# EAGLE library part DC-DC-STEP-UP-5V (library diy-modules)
DC/DC Step-Up Converter
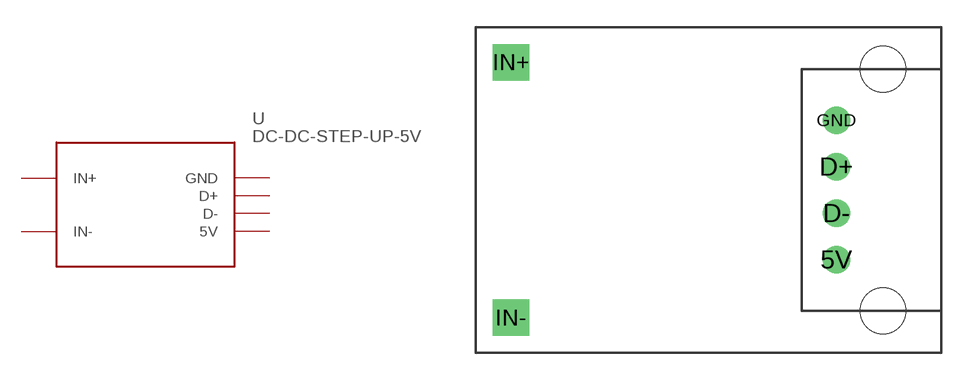
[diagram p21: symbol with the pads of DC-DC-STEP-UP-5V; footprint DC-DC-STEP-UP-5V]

Designator prefix -

## DC-DC-STEP-UP-5V  [DC-DC-STEP-UP-5V]
5V  5V
D+  D+
D-  D-
GND  GND
IN+  IN+  pwr
IN-  IN-  pwr

## Footprint DC-DC-STEP-UP-5V (pad centres in mm)
DC/DC Step-Up Converter
drill 1: 5V 6.985,-3.81; D+ 6.985,1.27; D- 6.985,-1.27; GND 6.985,3.81
drill 1 pad 2 square: IN+ -10.795,6.985; IN- -10.795,-6.985
hole 2.5 at 9.525,6.604
hole 2.5 at 9.525,-6.604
